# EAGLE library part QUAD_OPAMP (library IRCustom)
OP AMP Standard quad package
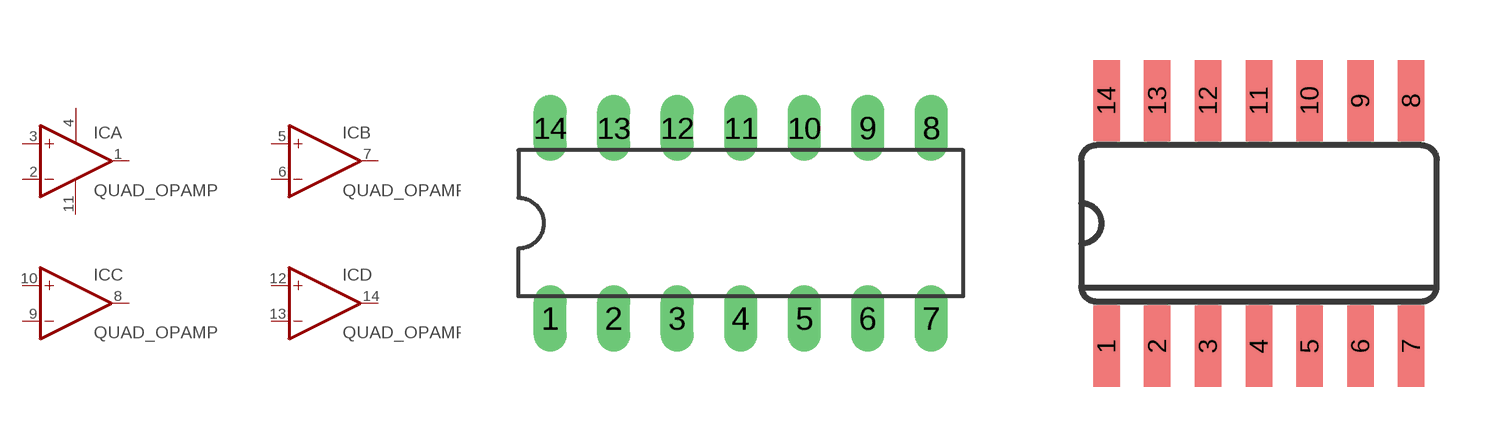
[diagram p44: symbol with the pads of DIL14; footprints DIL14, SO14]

Designator prefix IC; gates A=OPAMP B=OPAMP C=OPAMP D=OPAMP P=PWR+-

## QUAD_OPAMPP  [DIL14]
1  A:OUT  out
2  A:-IN  in
3  A:+IN  in
4  P:V+  pwr
5  B:+IN  in
6  B:-IN  in
7  B:OUT  out
8  C:OUT  out
9  C:-IN  in
10  C:+IN  in
11  P:V-  pwr
12  D:+IN  in
13  D:-IN  in
14  D:OUT  out

## QUAD_OPAMPD  [SO14]
Pads as for DIL14

## QUAD_OPAMPP-TI  [DIL14-LARDO]
Pads as for DIL14

## Footprint DIL14 (pad centres in mm)
Dual In Line Package
drill 0.813 long: 1 -7.62,-3.81; 2 -5.08,-3.81; 3 -2.54,-3.81; 4 0,-3.81; 5 2.54,-3.81; 6 5.08,-3.81; 7 7.62,-3.81; 8 7.62,3.81; 9 5.08,3.81; 10 2.54,3.81; 11 0,3.81; 12 -2.54,3.81; 13 -5.08,3.81; 14 -7.62,3.81

## Footprint SO14 (pad centres in mm)
Small Outline package 150 mil
smd 0.66 x 2.032: 1 -3.81,-3.073; 2 -2.54,-3.073; 3 -1.27,-3.073; 4 0,-3.073; 5 1.27,-3.073; 6 2.54,-3.073; 7 3.81,-3.073; 8 3.81,3.073; 9 2.54,3.073; 10 1.27,3.073; 11 0,3.073; 12 -1.27,3.073; 13 -2.54,3.073; 14 -3.81,3.073

## Footprint DIL14-LARDO (pad centres in mm)
drill 0.813 long: 1 -7.62,-3.81; 2 -5.08,-3.81; 3 -2.54,-3.81; 4 0,-3.81; 5 2.54,-3.81; 6 5.08,-3.81; 7 7.62,-3.81; 8 7.62,3.81; 9 5.08,3.81; 10 2.54,3.81; 11 0,3.81; 12 -2.54,3.81; 13 -5.08,3.81; 14 -7.62,3.81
